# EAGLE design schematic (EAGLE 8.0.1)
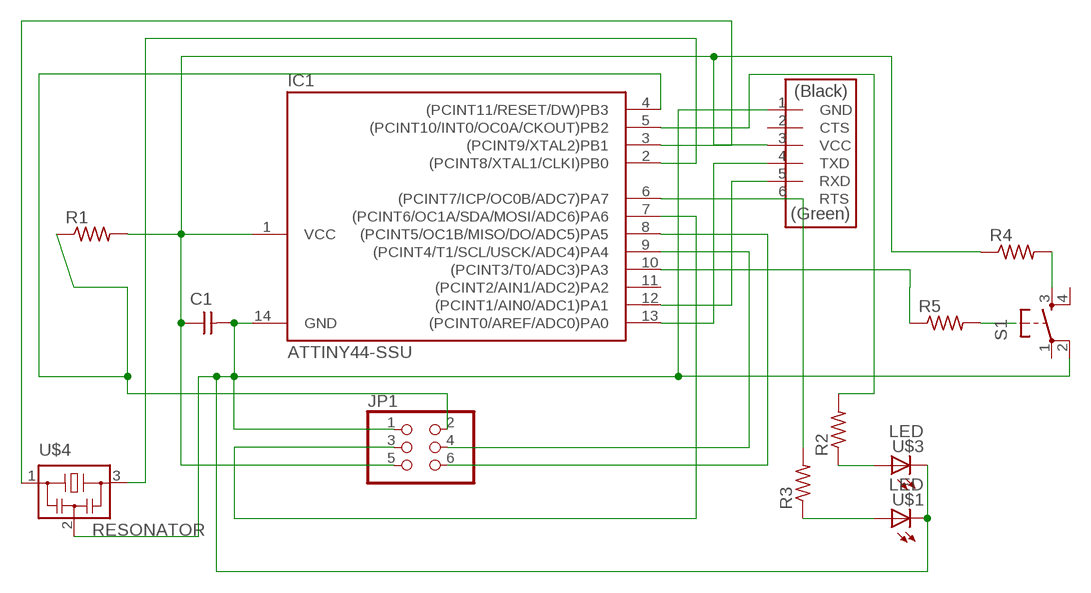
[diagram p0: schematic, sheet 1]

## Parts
C1  CAP-UNPOLARIZED  [C1206]
IC1  ATTINY44-SSU  [SOIC14]
JP1  PINHD-2X3-SMD  [2X03SMD]
R1  RES-US1206  [R1206]
R2  RES-US1206  [R1206]
R3  RES-US1206  [R1206]
R4  RES-US1206  [R1206]
R5  RES-US1206FAB  [R1206FAB]
S1  6MM_SWITCH6MM_SWITCH  [6MM_SWITCH]
U$1  LED  [LED1206]
U$2  FTDI-SMD-HEADER  [1X06SMD]
U$3  LED  [LED1206]
U$4  RESONATOR  [EFOBM]

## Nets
N$1: C1.1 IC1.1(VCC) JP1.5 R1.2 R4.1 U$2.3(VCC)
N$2: IC1.5((PCINT10/INT0/OC0A/CKOUT)PB2) R2.2
N$3: IC1.7((PCINT6/OC1A/SDA/MOSI/ADC6)PA6) JP1.3
N$4: IC1.13((PCINT0/AREF/ADC0)PA0) U$2.4(TXD)
N$5: IC1.12((PCINT1/AIN0/ADC1)PA1) U$2.5(RXD)
N$6: IC1.4((PCINT11/RESET/DW)PB3) JP1.2 R1.1
N$7: IC1.9((PCINT4/T1/SCL/USCK/ADC4)PA4) JP1.4
N$8: IC1.8((PCINT5/OC1B/MISO/DO/ADC5)PA5) JP1.6
N$9: R2.1 U$3.1(A)
N$10: IC1.2((PCINT8/XTAL1/CLKI)PB0) U$4.3
N$11: IC1.3((PCINT9/XTAL2)PB1) U$4.1
N$12: R3.1 U$1.1(A)
N$13: C1.2 IC1.14(GND) JP1.1 S1.2(P1) U$1.2(C) U$2.1(GND) U$3.2(C) U$4.2
N$14: IC1.6((PCINT7/ICP/OC0B/ADC7)PA7) R3.2
N$16: R4.2 S1.3(S)
N$17: IC1.10((PCINT3/T0/ADC3)PA3) R5.1
N$18: R5.2
Unconnected: IC1.11((PCINT2/AIN1/ADC2)PA2) S1.1(P) S1.4(S1) U$2.2(CTS) U$2.6(RTS)

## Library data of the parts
C1 = fab:CAP-UNPOLARIZED
IC1 = fab:ATTINY44
JP1 = fab:PINHD-2X3-SMD: PIN HEADER
R1-R5 = fab:RES-US: Resistor (US Symbol)
S1 = fab:6MM_SWITCH: OMRON SWITCH
U$1 U$3 = fab:LED: LED
U$2 = fab:FTDI-SMD-HEADER
U$4 = fab:RESONATOR

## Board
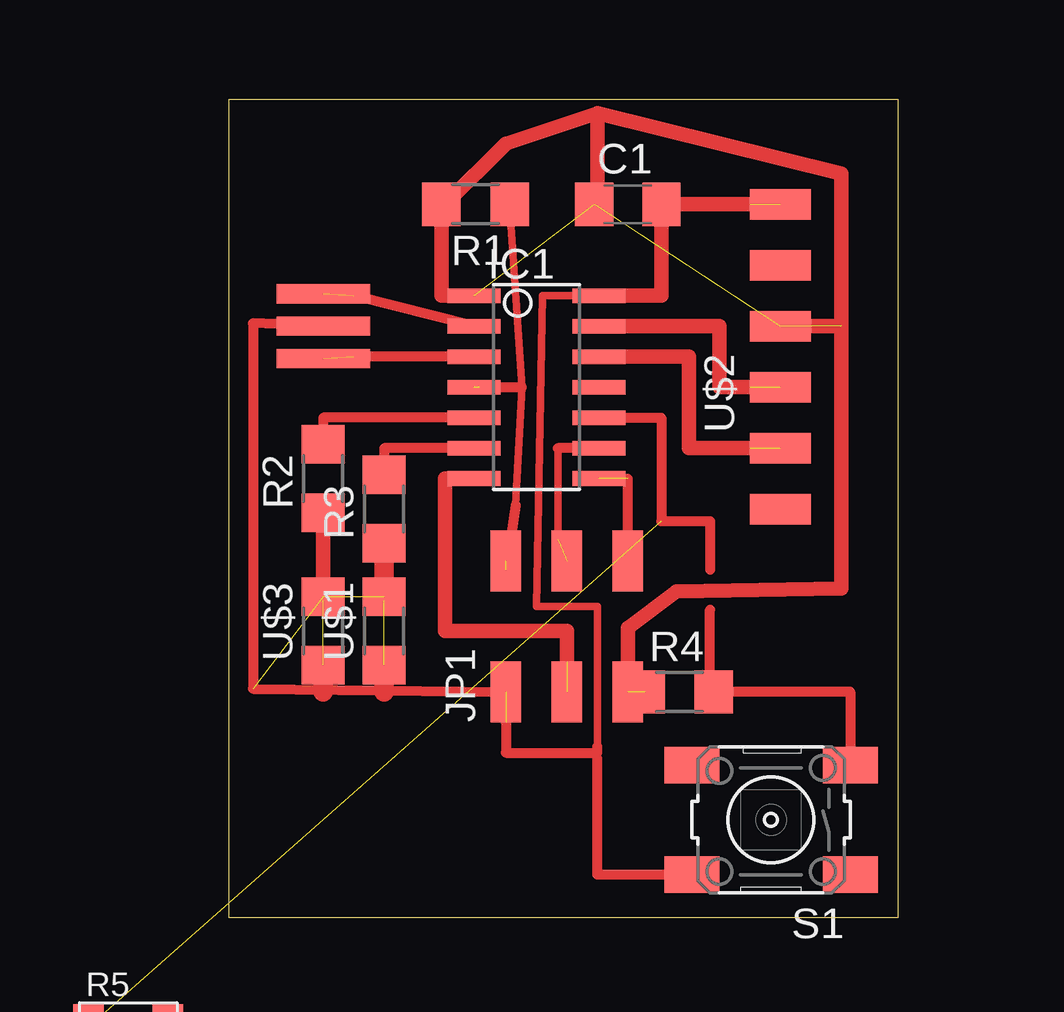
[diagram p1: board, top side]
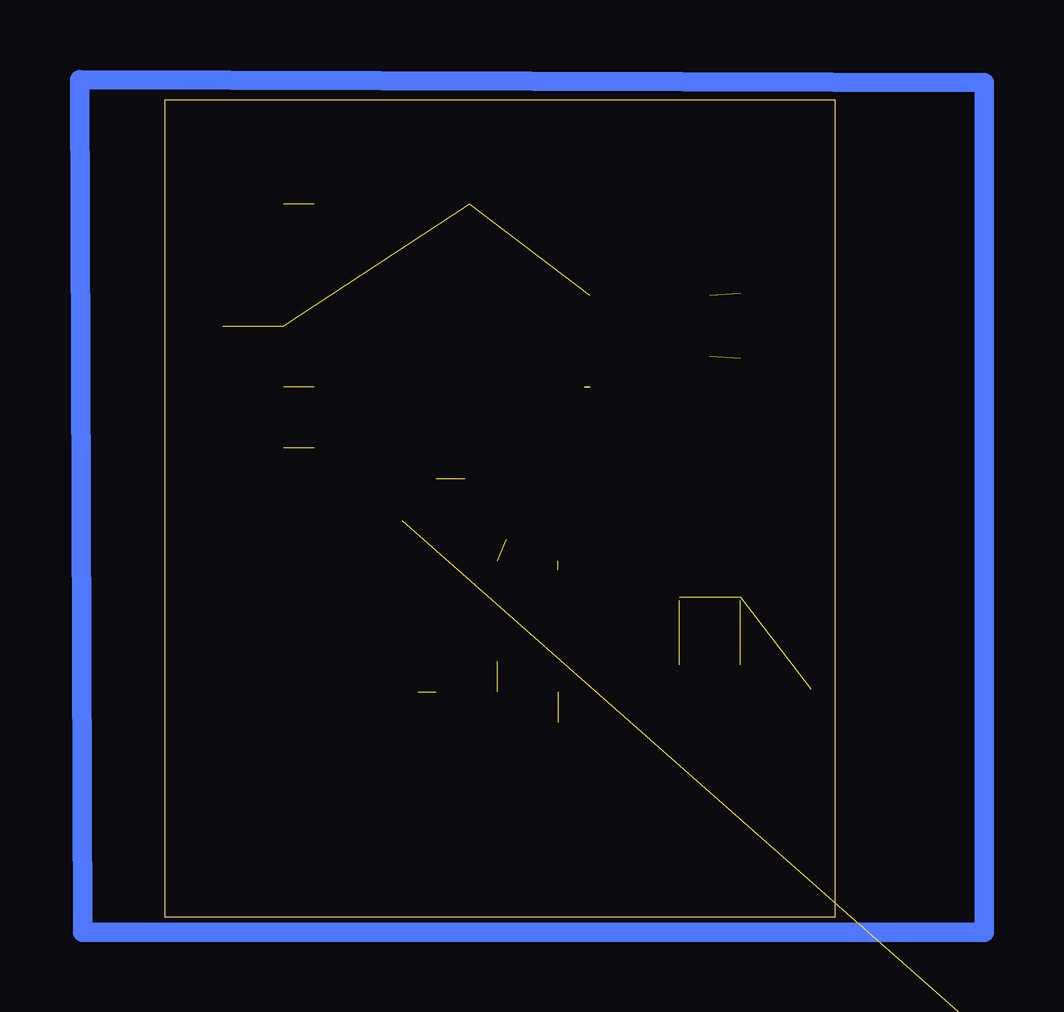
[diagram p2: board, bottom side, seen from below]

Size 27.92 x 34.09 mm. Coordinates in mm from the lower left corner, seen from the top.
Outline: 0,0 27.92,0 27.92,34.09 0,34.09 0,0
Copper layers (1*16): Top 0.035mm / dielectric 1.5mm / Bottom 0.035mm
Design rules "default": minimum track width 10mil, minimum drill 24mil, track to track 8mil, track to pad 8mil, pad to pad 8mil, via to via 8mil, smd to smd 8mil, copper to edge 40mil, drill to drill 8mil, minimum pad ring 10mil, minimum via ring 8mil, stop-mask expansion 4mil, vias tented up to drill 0mil, thermal gap 10mil

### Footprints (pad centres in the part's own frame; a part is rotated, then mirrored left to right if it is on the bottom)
C1206 = smd 1.6 x 1.8: 1 -1.4,0; 2 1.4,0
SOIC14 = smd 0.61 x 2.21: 1 -3.81,-2.603; 2 -2.54,-2.603; 3 -1.27,-2.603; 4 0,-2.603; 5 1.27,-2.603; 6 2.54,-2.603; 7 3.81,-2.603; 8 3.81,2.603; 9 2.54,2.603; 10 1.27,2.603; 11 0,2.603; 12 -1.27,2.603; 13 -2.54,2.603; 14 -3.81,2.603
2X03SMD = smd 2.54 x 1.27: 1 -2.54,2.54; 2 2.92,2.54; 3 -2.54,0; 4 2.92,0; 5 -2.54,-2.54; 6 2.92,-2.54
R1206 = smd 1.6 x 1.803: 1 -1.422,0; 2 1.422,0
R1206FAB = smd 1.27 x 1.905: 1 -1.651,0; 2 1.651,0
6MM_SWITCH = smd 2.286 x 1.524: 1 -3.302,2.286; 2 3.302,2.286; 3 -3.302,-2.286; 4 3.302,-2.286
LED1206 = smd 1.6 x 1.803: 1 -1.422,0; 2 1.422,0
1X06SMD = smd 2.54 x 1.27: 1 0,6.35; 2 0,3.81; 3 0,1.27; 4 0,-1.27; 5 0,-3.81; 6 0,-6.35
EFOBM = smd 0.8 x 3.9: 1 -1.35,0; 2 0,0; 3 1.35,0

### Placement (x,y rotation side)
C1  16.64,29.72 0 top
IC1  12.83,22.1 270 top
JP1  14.1,11.94 90 top
R1  10.29,29.72 180 top
R2  3.94,18.29 90 top
R3  6.48,17.02 90 top
R4  18.8,9.4 0 top
R5  not placed on the board
S1  22.61,4.06 180 top
U$1  6.48,11.94 90 top
U$2  22.99,23.37 0 top
U$3  3.94,11.94 90 top
U$4  3.94,24.64 90 top

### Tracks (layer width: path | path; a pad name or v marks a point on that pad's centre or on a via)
N$1  (4 unrouted)
  Top 0.61: IC1.1 8.87,25.91 R1.2 | JP1.5 16.64,12.06 18.67,13.59 25.53,13.72 25.53,24.64
N$2
  Top 0.406: IC1.5 3.94,20.83 R2.2
N$3  (1 unrouted)
  Top 0.61: IC1.7 9.02,18.29 9.02,11.94 14.1,11.94 14.1,10.67
N$4  (1 unrouted)
  Top 0.61: IC1.13 20.45,24.64 20.45,22.1 21.72,22.1
N$5  (1 unrouted)
  Top 0.61: IC1.12 19.18,23.37 19.18,19.56 21.72,19.56
N$6  (3 unrouted)
  Top 0.305: R1.1 12.22,22.1 11.96,17.17
  Top 0.406: 11.96,17.17 11.56,14.48 | 9.53,22.1 IC1.4 12.22,22.1
N$7  (1 unrouted)
  Top 0.305: 13.72,19.56 13.72,15.75
  Top 0.406: IC1.9 13.72,19.56
N$8  (1 unrouted)
  Top 0.406: JP1.6 16.64,18.29
N$9  (1 unrouted)
  Top 0.61: R2.1 3.94,13.21
  Top 0.813: U$3.1 3.94,9.4
N$10  (1 unrouted)
  Top 0.406: IC1.2 5.21,25.91
N$11  (1 unrouted)
  Top 0.406: IC1.3 5.21,23.37
N$12  (1 unrouted)
  Top 0.813: R3.1 6.48,13.21 | U$1.1 6.48,9.4
N$13  (4 unrouted)
  Top 0.305: IC1.14 13.08,25.91 12.83,12.95 15.37,12.95 15.37,7.11 15.37,6.6
  Top 0.406: 11.56,8.13 11.56,6.86 15.37,6.86 15.37,7.11 | U$4.2 1.02,24.77 1.02,9.52 JP1.1 | S1.2 15.37,1.78 15.37,6.6
  Top 0.61: 21.72,29.72 C1.2 18.04,25.91 IC1.14
N$14
  Top 0.406: IC1.6 6.48,19.56 R3.2
N$15
  Bottom 0.813: -6.22,34.8 31.5,34.92 31.37,-0.64 -6.22,-0.64 -6.22,34.8
N$16
  Top 0.406: S1.3 25.91,9.4 R4.2 20.07,9.4 20.07,12.83
  Top 0.813: R4.2 20.19,9.4 20.19,9.65
N$17  (1 unrouted)
  Top 0.406: IC1.10 18.03,20.83 18.03,16.51 20.07,16.51 20.07,14.48
VCC
  Top 0.61: 15.37,29.72 15.37,33.53 | 15.37,33.53 25.53,30.99 25.53,24.64 22.99,24.64 | 15.37,33.53 11.56,32.26 9.02,29.72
